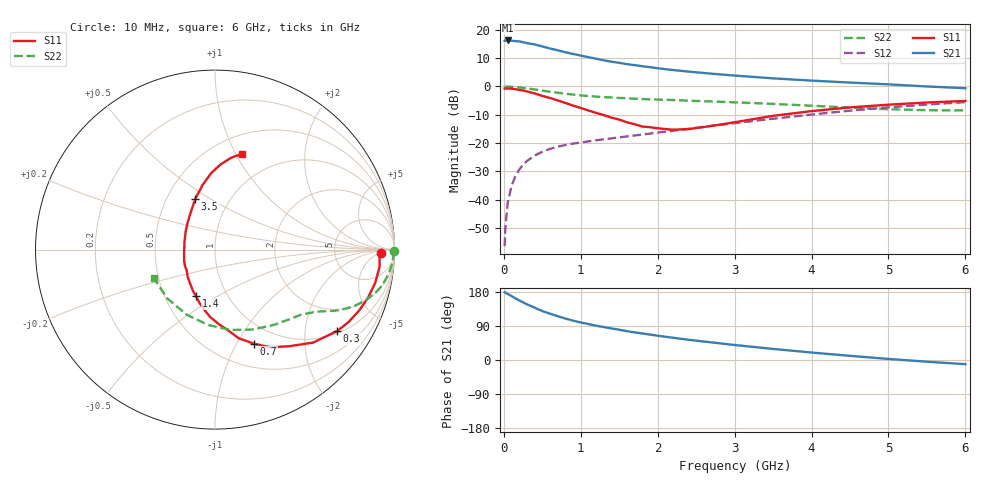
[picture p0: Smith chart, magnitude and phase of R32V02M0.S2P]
! SIEMENS Small Signal Semiconductors
! BFR181
! Si NPN RF Bipolar Junction Transistor in SOT23
! VCE = 2 V  IC = 2 mA
! Common Emitter S-Parameters:  May  1996
# GHz  S  MA  R  50
!  f  S11  S21  S12  S22
! GHz  MAG  ANG  MAG  ANG  MAG  ANG  MAG  ANG
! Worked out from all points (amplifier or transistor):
!   36 points, 10 MHz to 6 GHz, reference 50 ohm
!   highest |S21| = 16.3 dB at 50 MHz (marker M1)
!   |S21| within 3 dB of that: start of sweep to 626.8 MHz
!   unconditionally stable (mu >= 1): 1.563 GHz to 3.378 GHz
!   at 250 MHz: K = 0.24, MSG = 21.7 dB, |S12| = -27.7 dB
!   at 1.4 GHz: K = 0.95, MSG = 13.6 dB, |S12| = -18.4 dB
!   at 6 GHz: K = 0.87, MSG = 2.5 dB, |S12| = -5.6 dB
!   lowest NFmin = 1.35 dB at 450 MHz
!   S11 on the Smith chart (normalised r, x): 10 MHz: 24, -7; 300 MHz: 1.08, -2.95; 700 MHz: 0.76, -1.18; 1.4 GHz: 0.71, -0.40; 3.5 GHz: 0.69, +0.43; 6 GHz: 0.69, +1.06
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0.01  0.9245 -1.3  6.463 179.1  0.0015 100.6  0.997 -0.6
0.02  0.917 -2.0  6.361 177.6  0.0032 86.6  0.9945 -1.1
0.05  0.9223 -6.0  6.506 174.3  0.0087 84.4  0.9937 -2.7
0.1  0.9113 -11.8  6.461 168.9  0.0175 83.3  0.9868 -5.5
0.15  0.8937 -17.5  6.329 162.5  0.0259 79.5  0.9767 -8.1
0.2  0.872 -22.9  6.266 157.3  0.0339 76.9  0.9617 -10.5
0.3  0.8178 -33.7  5.846 146.9  0.048 70.6  0.9264 -15.0
0.4  0.753 -43.5  5.535 138.1  0.0601 66.0  0.886 -18.6
0.5  0.6806 -52.2  5.093 129.0  0.07 62.0  0.8438 -21.6
0.7  0.5666 -67.6  4.361 115.7  0.0859 56.7  0.7743 -25.8
0.8  0.5108 -75.1  4.026 109.4  0.0923 54.9  0.7451 -27.2
0.9  0.4589 -80.4  3.757 103.8  0.0977 53.9  0.7185 -28.5
1.1  0.3761 -94.2  3.299 94.8  0.107 53.0  0.6773 -30.6
1.2  0.3406 -100.0  3.092 90.5  0.1117 52.8  0.6613 -31.7
1.4  0.2807 -112.2  2.739 83.2  0.1208 52.8  0.6376 -33.6
1.7  0.2148 -135.1  2.38 72.9  0.1358 53.7  0.6073 -36.2
2.2  0.1716 -178.6  1.951 58.7  0.1649 55.1  0.5748 -42.0
2.8  0.2102 137.3  1.64 44.2  0.2085 55.3  0.5369 -50.7
3.5  0.3023 111.4  1.391 29.2  0.2687 52.7  0.4915 -64.9
4.5  0.4264 92.9  1.171 11.0  0.3732 44.4  0.4218 -95.1
5.5  0.5205 79.9  1 -4.5  0.4794 31.9  0.3804 -134.2
6  0.5549 74.1  0.931 -11.0  0.5278 24.5  0.3763 -155.0
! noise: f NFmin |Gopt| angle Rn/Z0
0.45  1.35  0.6  17  0.4
0.9  1.45  0.5  36  0.4
1.8  1.8  0.31  80  0.37
